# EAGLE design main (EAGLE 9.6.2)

## Sheet 1 of 4: Anschluesse
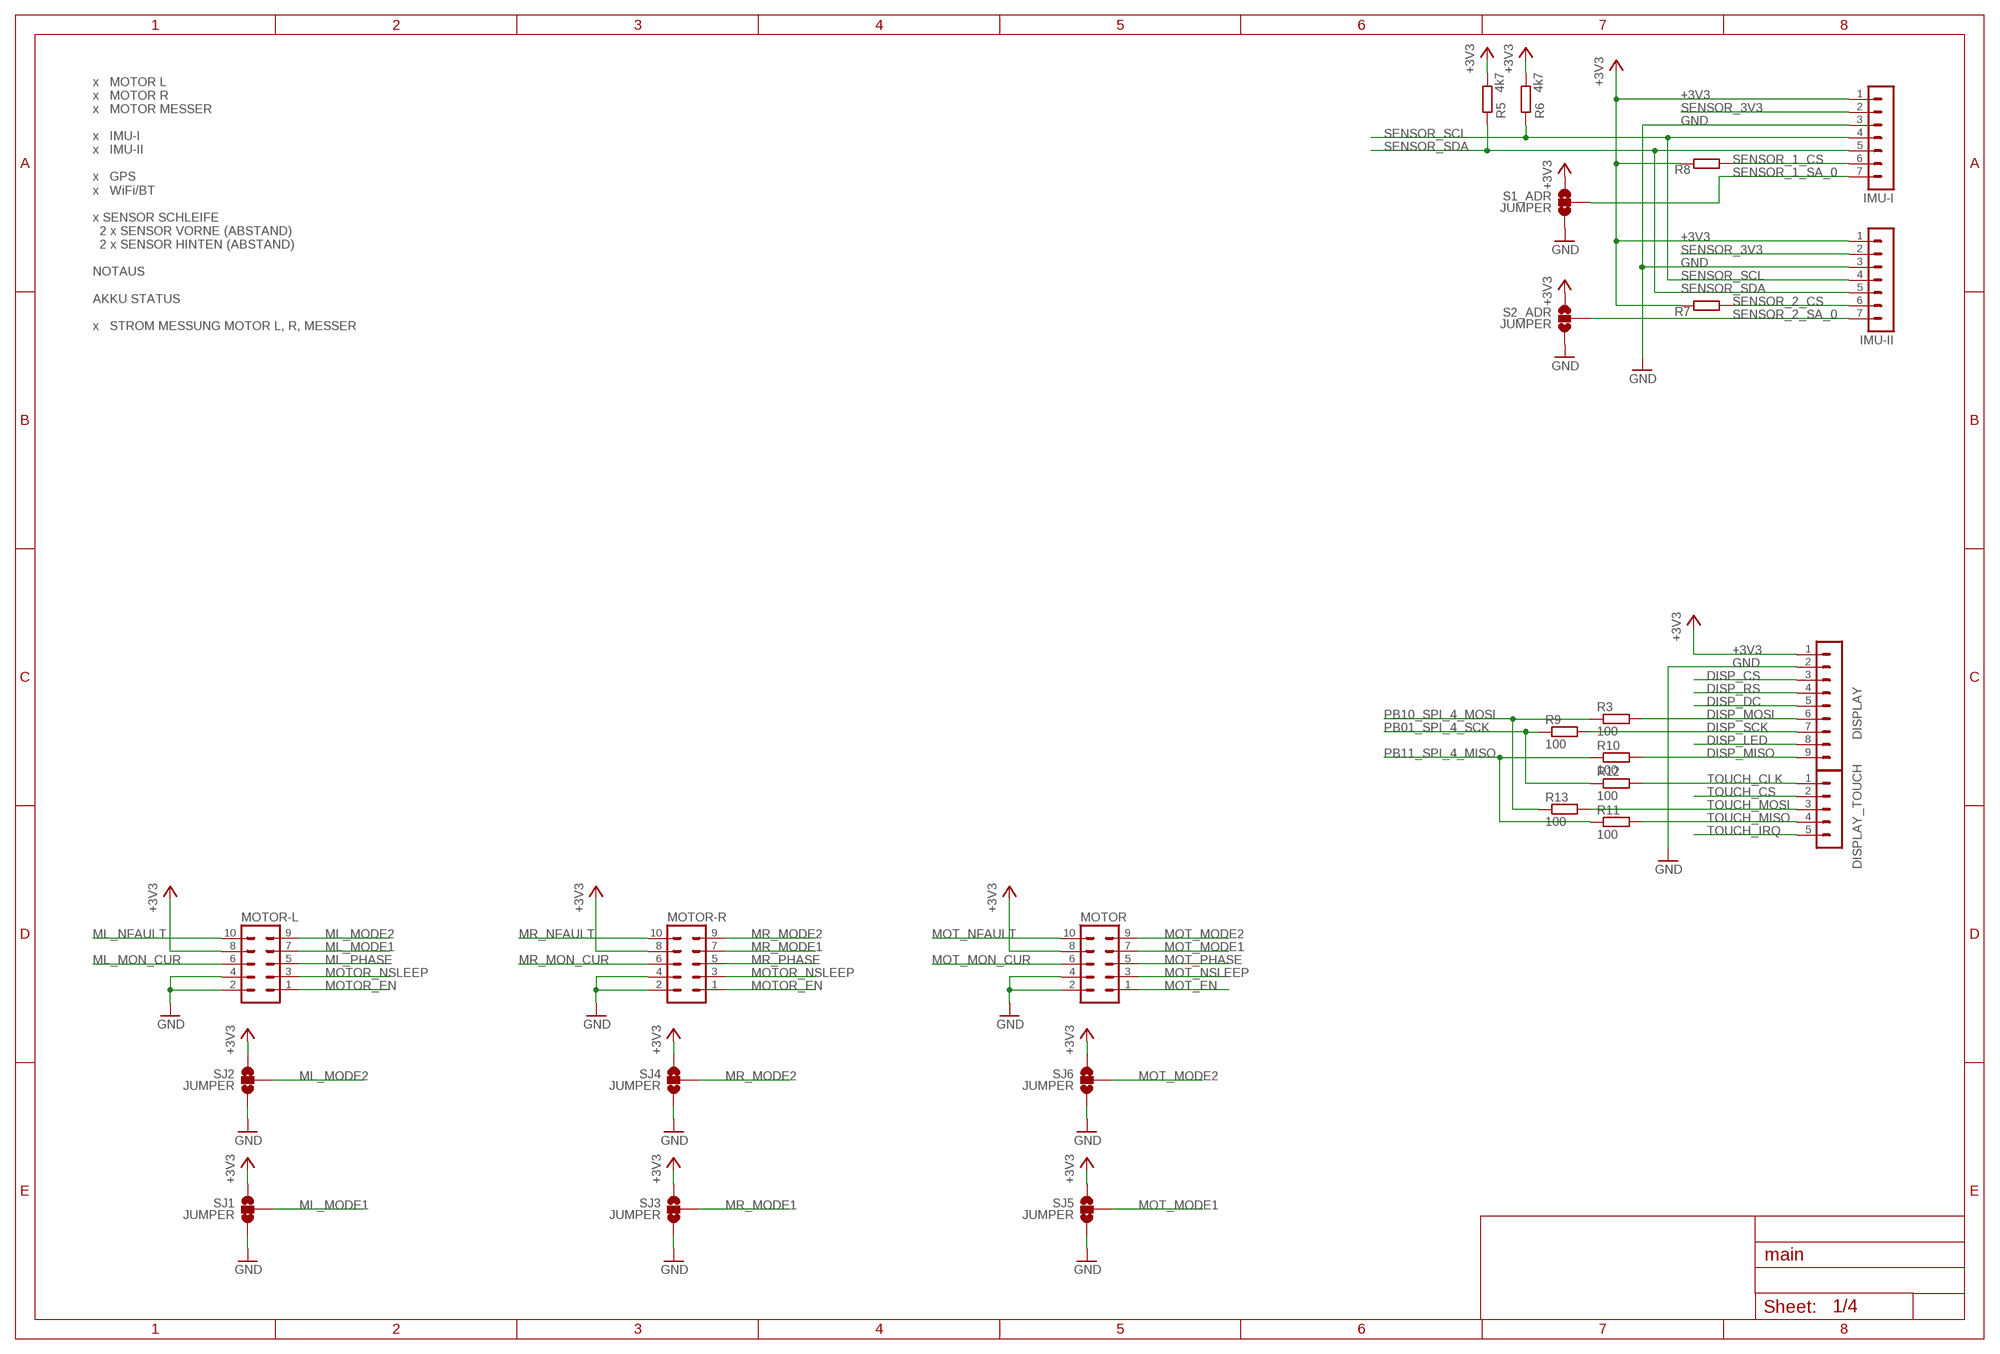
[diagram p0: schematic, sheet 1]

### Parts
DISPLAY  MA09-1  [MA09-1]
DISPLAY_TOUCH  MA05-1  [MA05-1]
IMU-I  MA07-1  [MA07-1]
IMU-II  MA07-1  [MA07-1]
MOTOR  ML10  [ML10]
MOTOR-L  ML10  [ML10]
MOTOR-R  ML10  [ML10]
R3  100  R-EU_R0603  [R0603]
R5  4k7  R-EU_R0603  [R0603]
R6  4k7  R-EU_R0603  [R0603]
R7  R-EU_R0603  [R0603]
R8  R-EU_R0603  [R0603]
R9  100  R-EU_R0603  [R0603]
R10  100  R-EU_R0603  [R0603]
R11  100  R-EU_R0603  [R0603]
R12  100  R-EU_R0603  [R0603]
R13  100  R-EU_R0603  [R0603]
S1_ADR  JUMPER  JUMPER-PAD-3-NOYES_SILK  [PAD-JUMPER-3-NO_YES_SILK]
S2_ADR  JUMPER  JUMPER-PAD-3-NOYES_SILK  [PAD-JUMPER-3-NO_YES_SILK]
SJ1  JUMPER  JUMPER-PAD-3-NOYES_SILK  [PAD-JUMPER-3-NO_YES_SILK]
SJ2  JUMPER  JUMPER-PAD-3-NOYES_SILK  [PAD-JUMPER-3-NO_YES_SILK]
SJ3  JUMPER  JUMPER-PAD-3-NOYES_SILK  [PAD-JUMPER-3-NO_YES_SILK]
SJ4  JUMPER  JUMPER-PAD-3-NOYES_SILK  [PAD-JUMPER-3-NO_YES_SILK]
SJ5  JUMPER  JUMPER-PAD-3-NOYES_SILK  [PAD-JUMPER-3-NO_YES_SILK]
SJ6  JUMPER  JUMPER-PAD-3-NOYES_SILK  [PAD-JUMPER-3-NO_YES_SILK]

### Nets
+3V3: DISPLAY.1 IMU-I.1 IMU-II.1 MOTOR-L.8 MOTOR-R.8 MOTOR.8 R5.2 R6.2 R7.2 R8.2 S1_ADR.1 S2_ADR.1 SJ1.1 SJ2.1 SJ3.1 SJ4.1 SJ5.1 SJ6.1 ; also sheet 2,3
DISP_CS: DISPLAY.3 ; also sheet 2
DISP_DC: DISPLAY.5 ; also sheet 2
DISP_LED: DISPLAY.8
DISP_MISO: DISPLAY.9 R10.2
DISP_MOSI: DISPLAY.6 R3.2
DISP_RS: DISPLAY.4 ; also sheet 2
DISP_SCK: DISPLAY.7 R9.2
GND: DISPLAY.2 IMU-I.3 IMU-II.3 MOTOR-L.2 MOTOR-L.4 MOTOR-R.2 MOTOR-R.4 MOTOR.2 MOTOR.4 S1_ADR.3 S2_ADR.3 SJ1.3 SJ2.3 SJ3.3 SJ4.3 SJ5.3 SJ6.3 ; also sheet 2,3,4
ML_MODE1: MOTOR-L.7 SJ1.2
ML_MODE2: MOTOR-L.9 SJ2.2
ML_MON_CUR: MOTOR-L.6 ; also sheet 2
ML_NFAULT: MOTOR-L.10 ; also sheet 2
ML_PHASE: MOTOR-L.5 ; also sheet 2
MOT_EN: MOTOR.1 ; also sheet 2
MOT_MODE1: MOTOR.7 SJ5.2
MOT_MODE2: MOTOR.9 SJ6.2
MOT_MON_CUR: MOTOR.6 ; also sheet 2
MOT_NFAULT: MOTOR.10 ; also sheet 2
MOT_NSLEEP: MOTOR.3 ; also sheet 2
MOT_PHASE: MOTOR.5 ; also sheet 2
MOTOR_EN: MOTOR-L.1 MOTOR-R.1 ; also sheet 2
MOTOR_NSLEEP: MOTOR-L.3 MOTOR-R.3 ; also sheet 2
MR_MODE1: MOTOR-R.7 SJ3.2
MR_MODE2: MOTOR-R.9 SJ4.2
MR_MON_CUR: MOTOR-R.6 ; also sheet 2
MR_NFAULT: MOTOR-R.10 ; also sheet 2
MR_PHASE: MOTOR-R.5 ; also sheet 2
PB01_SPI_4_SCK: R9.1 R12.1 ; also sheet 2
PB10_SPI_4_MOSI: R3.1 R13.1 ; also sheet 2
PB11_SPI_4_MISO: R10.1 R11.1 ; also sheet 2
SENSOR_1_CS: IMU-I.6 R8.1
SENSOR_1_SA_0: IMU-I.7 S1_ADR.2
SENSOR_2_CS: IMU-II.6 R7.1
SENSOR_2_SA_0: IMU-II.7 S2_ADR.2
SENSOR_3V3: IMU-I.2 IMU-II.2
SENSOR_SCL: IMU-I.4 IMU-II.4 R6.1 ; also sheet 2
SENSOR_SDA: IMU-I.5 IMU-II.5 R5.1 ; also sheet 2
TOUCH_CLK: DISPLAY_TOUCH.1 R12.2
TOUCH_CS: DISPLAY_TOUCH.2 ; also sheet 2
TOUCH_IRQ: DISPLAY_TOUCH.5 ; also sheet 2
TOUCH_MISO: DISPLAY_TOUCH.4 R11.2
TOUCH_MOSI: DISPLAY_TOUCH.3 R13.2

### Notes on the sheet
- x   MOTOR L
  x   MOTOR R
  x   MOTOR MESSER
  
  x   IMU-I
  x   IMU-II
  
  x   GPS
  x   WiFi/BT
  
  x SENSOR SCHLEIFE
    2 x SENSOR VORNE (ABSTAND)
    2 x SENSOR HINTEN (ABSTAND)
  
  NOTAUS
  
  AKKU STATUS
  
  x   STROM MESSUNG MOTOR L, R, MESSER

## Sheet 2 of 4: CPU
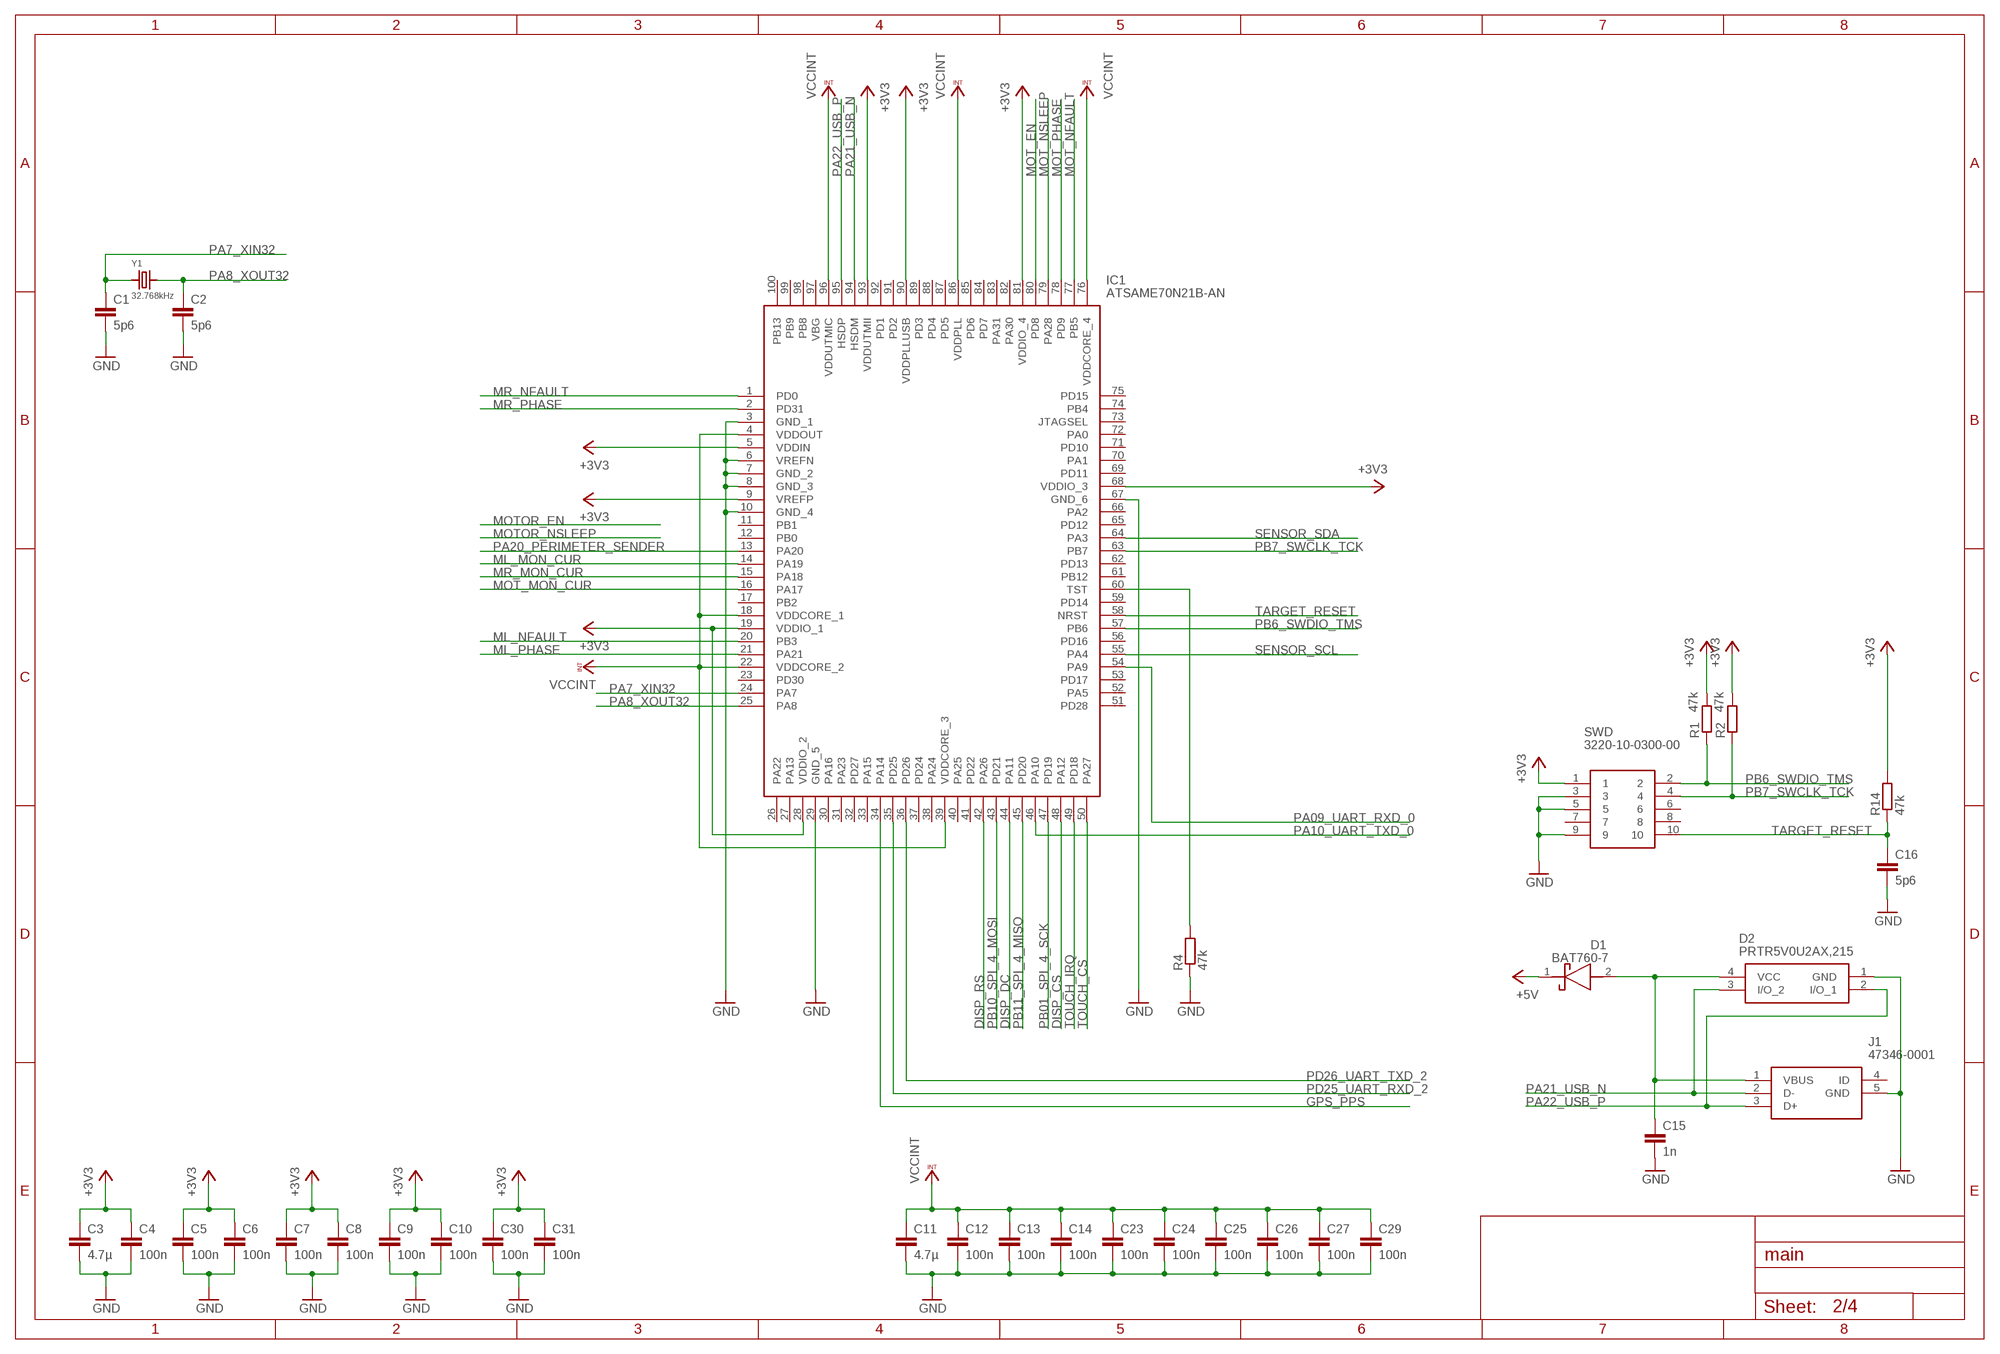
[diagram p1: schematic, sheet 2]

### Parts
C1  5p6  C-EUC0603  [C0603]
C2  5p6  C-EUC0603  [C0603]
C3  4.7µ  C-EUC0603  [C0603]
C4  100n  C-EUC0603  [C0603]
C5  100n  C-EUC0603  [C0603]
C6  100n  C-EUC0603  [C0603]
C7  100n  C-EUC0603  [C0603]
C8  100n  C-EUC0603  [C0603]
C9  100n  C-EUC0603  [C0603]
C10  100n  C-EUC0603  [C0603]
C11  4.7µ  C-EUC0603  [C0603]
C12  100n  C-EUC0603  [C0603]
C13  100n  C-EUC0603  [C0603]
C14  100n  C-EUC0603  [C0603]
C15  1n  C-EUC0603  [C0603]
C16  5p6  C-EUC0603  [C0603]
C23  100n  C-EUC0603  [C0603]
C24  100n  C-EUC0603  [C0603]
C25  100n  C-EUC0603  [C0603]
C26  100n  C-EUC0603  [C0603]
C27  100n  C-EUC0603  [C0603]
C29  100n  C-EUC0603  [C0603]
C30  100n  C-EUC0603  [C0603]
C31  100n  C-EUC0603  [C0603]
D1  BAT760-7  [SOD2513X120N]
D2  PRTR5V0U2AX,215  [PESD2ETHAXR]
IC1  ATSAME70N21B-AN  [QFP50P1600X1600X160-100N]
J1  47346-0001  [47346-0001]
R1  47k  R-EU_R0603  [R0603]
R2  47k  R-EU_R0603  [R0603]
R4  47k  R-EU_R0603  [R0603]
R14  47k  R-EU_R0603  [R0603]
SWD  3220-10-0300-00  [3220-10-0300-00]
Y1  32.768kHz  CRYSTALTHIN32K  [CRYSTAL_4.9X1.8]

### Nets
+3V3: C3.1 C4.1 C5.1 C6.1 C7.1 C8.1 C9.1 C10.1 C30.1 C31.1 IC1.5(VDDIN) IC1.9(VREFP) IC1.19(VDDIO_1) IC1.28(VDDIO_2) IC1.68(VDDIO_3) IC1.81(VDDIO_4) IC1.90(VDDPLLUSB) IC1.93(VDDUTMII) R1.2 R2.2 R14.2 SWD.1 ; also sheet 1,3
+5V: D1.1(K) ; also sheet 4
DISP_CS: IC1.48(PA12) ; also sheet 1
DISP_DC: IC1.44(PA11) ; also sheet 1
DISP_RS: IC1.42(PA26) ; also sheet 1
GND: C1.2 C2.2 C3.2 C4.2 C5.2 C6.2 C7.2 C8.2 C9.2 C10.2 C11.2 C12.2 C13.2 C14.2 C15.2 C16.2 C23.2 C24.2 C25.2 C26.2 C27.2 C29.2 C30.2 C31.2 D2.1(GND) IC1.3(GND_1) IC1.6(VREFN) IC1.7(GND_2) IC1.8(GND_3) IC1.10(GND_4) IC1.29(GND_5) IC1.67(GND_6) J1.5(GND) R4.1 SWD.3 SWD.5 SWD.9 ; also sheet 1,3,4
GPS_PPS: IC1.34(PA14) ; also sheet 3
ML_MON_CUR: IC1.14(PA19) ; also sheet 1
ML_NFAULT: IC1.20(PB3) ; also sheet 1
ML_PHASE: IC1.21(PA21) ; also sheet 1
MOT_EN: IC1.80(PD8) ; also sheet 1
MOT_MON_CUR: IC1.16(PA17) ; also sheet 1
MOT_NFAULT: IC1.77(PB5) ; also sheet 1
MOT_NSLEEP: IC1.79(PA28) ; also sheet 1
MOT_PHASE: IC1.78(PD9) ; also sheet 1
MR_MON_CUR: IC1.15(PA18) ; also sheet 1
MR_NFAULT: IC1.1(PD0) ; also sheet 1
MR_PHASE: IC1.2(PD31) ; also sheet 1
N$1: IC1.60(TST) R4.2
N$2: C15.1 D1.2(A) D2.4(VCC) J1.1(VBUS)
PA7_XIN32: C1.1 IC1.24(PA7) Y1.1
PA8_XOUT32: C2.1 IC1.25(PA8) Y1.2
PA09_UART_RXD_0: IC1.54(PA9) ; also sheet 3
PA10_UART_TXD_0: IC1.46(PA10) ; also sheet 3
PA20_PERIMETER_SENDER: IC1.13(PA20) ; also sheet 4
PA21_USB_N: D2.3(I/O_2) IC1.94(HSDM) J1.2(D-)
PA22_USB_P: D2.2(I/O_1) IC1.95(HSDP) J1.3(D+)
PB01_SPI_4_SCK: IC1.47(PD19) ; also sheet 1
PB6_SWDIO_TMS: IC1.57(PB6) R1.1 SWD.2
PB7_SWCLK_TCK: IC1.63(PB7) R2.1 SWD.4
PB10_SPI_4_MOSI: IC1.43(PD21) ; also sheet 1
PB11_SPI_4_MISO: IC1.45(PD20) ; also sheet 1
PD25_UART_RXD_2: IC1.35(PD25) ; also sheet 3
PD26_UART_TXD_2: IC1.36(PD26) ; also sheet 3
SENSOR_SCL: IC1.55(PA4) ; also sheet 1
SENSOR_SDA: IC1.64(PA3) ; also sheet 1
TARGET_RESET: C16.1 IC1.58(NRST) R14.1 SWD.10
TOUCH_CS: IC1.50(PA27) ; also sheet 1
TOUCH_IRQ: IC1.49(PD18) ; also sheet 1
VCCINT: C11.1 C12.1 C13.1 C14.1 C23.1 C24.1 C25.1 C26.1 C27.1 C29.1 IC1.4(VDDOUT) IC1.18(VDDCORE_1) IC1.22(VDDCORE_2) IC1.39(VDDCORE_3) IC1.76(VDDCORE_4) IC1.86(VDDPLL) IC1.96(VDDUTMIC)
Unconnected: IC1.11(PB1) IC1.12(PB0) IC1.17(PB2) IC1.23(PD30) IC1.26(PA22) IC1.27(PA13) IC1.30(PA16) IC1.31(PA23) IC1.32(PD27) IC1.33(PA15) IC1.37(PD24) IC1.38(PA24) IC1.40(PA25) IC1.41(PD22) IC1.51(PD28) IC1.52(PA5) IC1.53(PD17) IC1.56(PD16) IC1.59(PD14) IC1.61(PB12) IC1.62(PD13) IC1.65(PD12) IC1.66(PA2) IC1.69(PD11) IC1.70(PA1) IC1.71(PD10) IC1.72(PA0) IC1.73(JTAGSEL) IC1.74(PB4) IC1.75(PD15) IC1.82(PA30) IC1.83(PA31) IC1.84(PD7) IC1.85(PD6) IC1.87(PD5) IC1.88(PD4) IC1.89(PD3) IC1.91(PD2) IC1.92(PD1) IC1.97(VBG) IC1.98(PB8) IC1.99(PB9) IC1.100(PB13) J1.4(ID) SWD.6 SWD.7 SWD.8

## Sheet 3 of 4: GPS WLAN BT
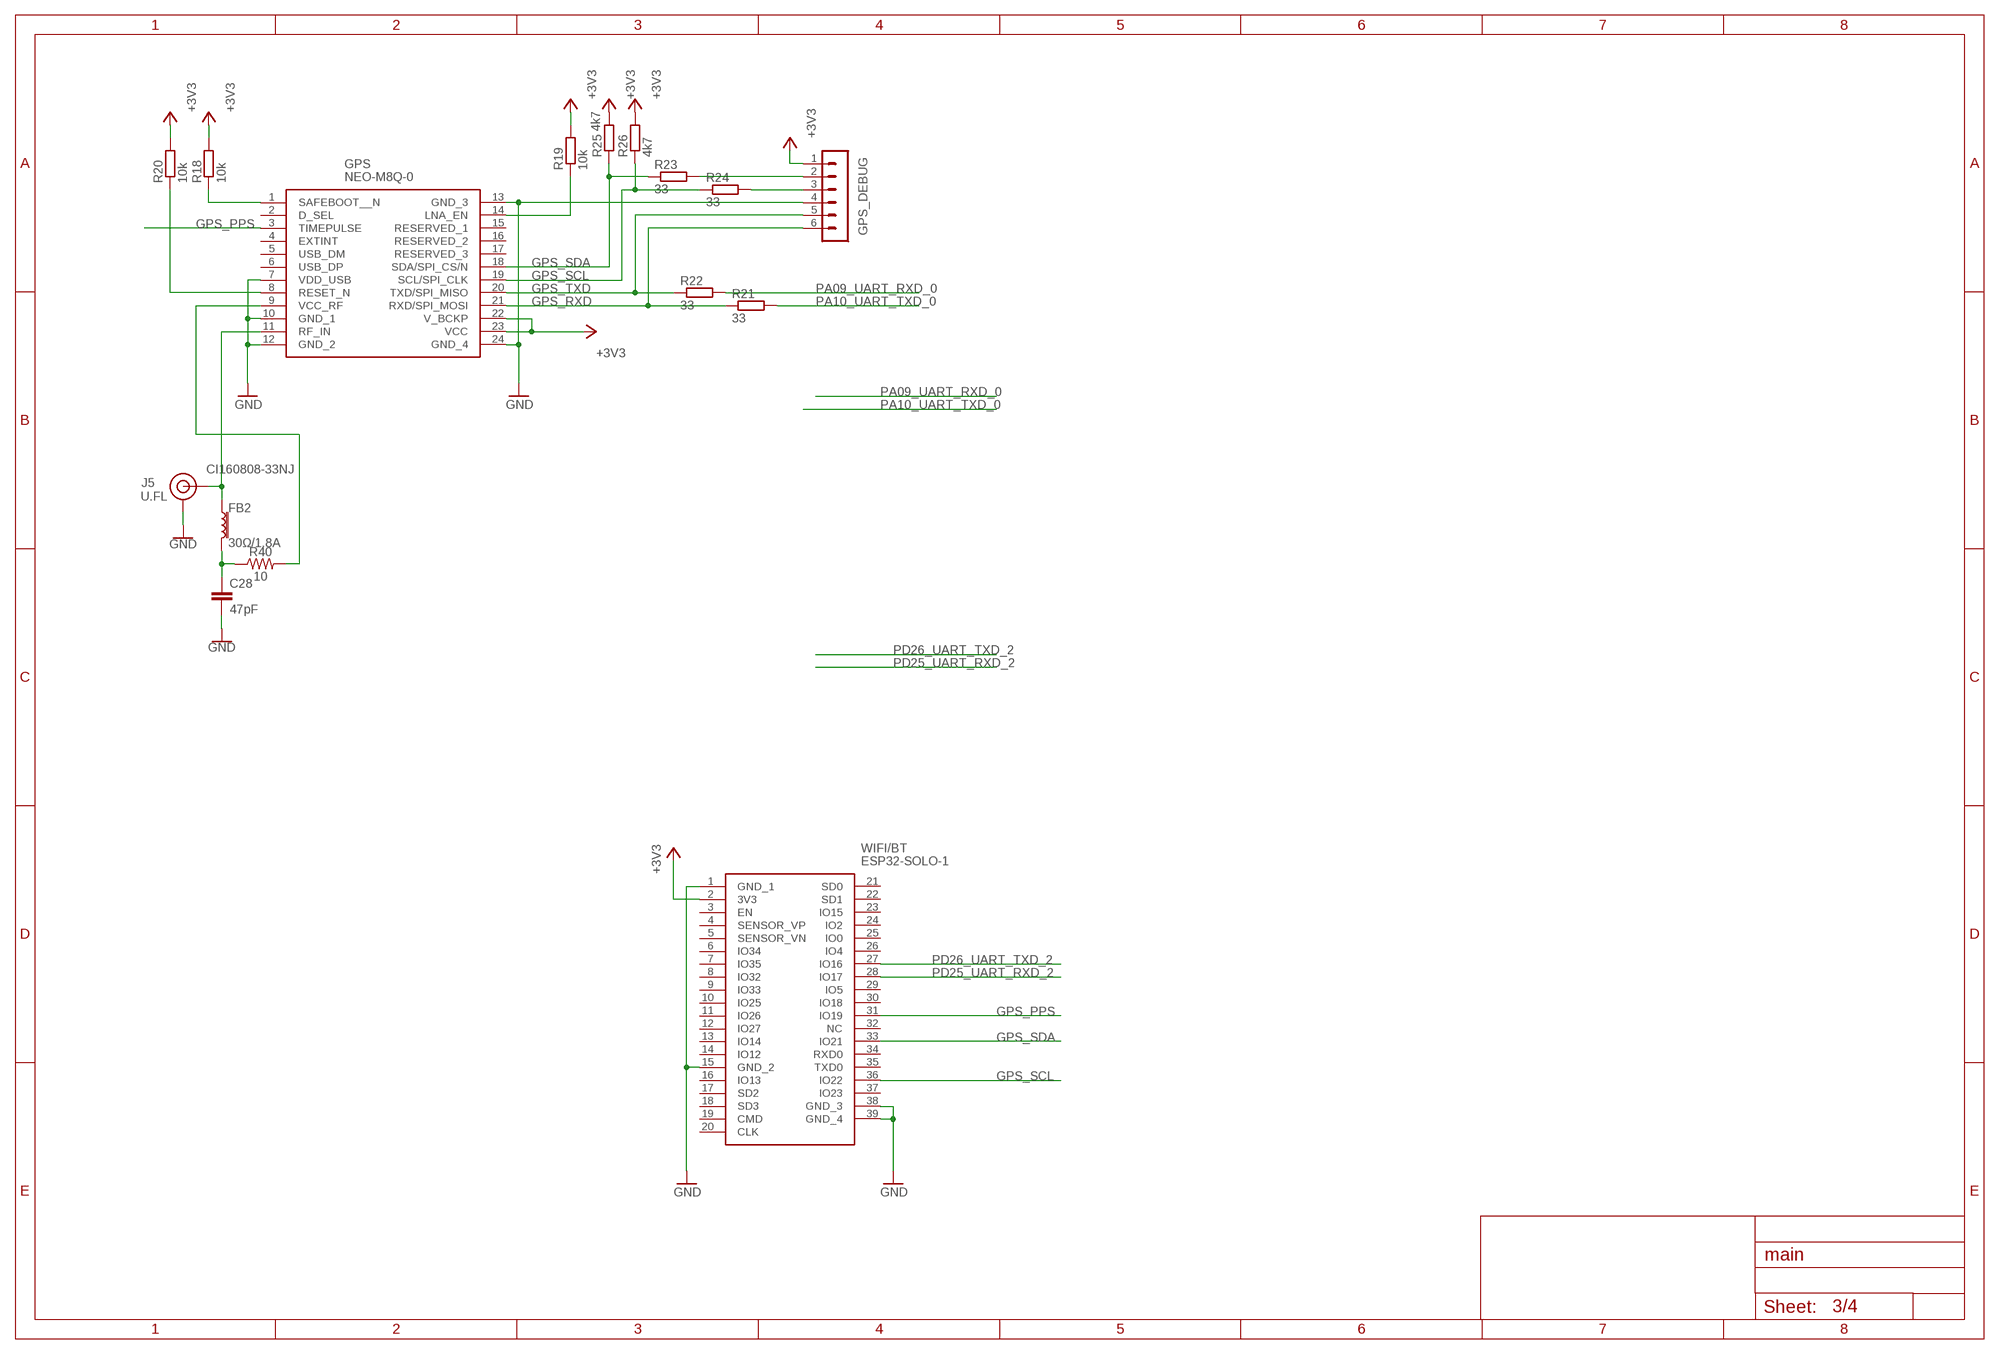
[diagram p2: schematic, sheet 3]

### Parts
C28  47pF  47PF-0603-50V-5%  [0603]
FB2  30Ω/1.8A  FERRITE_BEAD-0603  [0603]
GPS  NEO-M8Q-0  [NEO-M8U]
GPS_DEBUG  MA06-1  [MA06-1]
J5  U.FL  U.FL2PIN  [U.FL]
R18  10k  R-EU_R0603  [R0603]
R19  10k  R-EU_R0603  [R0603]
R20  10k  R-EU_R0603  [R0603]
R21  33  R-EU_R0603  [R0603]
R22  33  R-EU_R0603  [R0603]
R23  33  R-EU_R0603  [R0603]
R24  33  R-EU_R0603  [R0603]
R25  4k7  R-EU_R0603  [R0603]
R26  4k7  R-EU_R0603  [R0603]
R40  10  10OHM-0603-1/10W-1%  [0603]
WIFI/BT  ESP32-SOLO-1  [ESP32SOLO1]

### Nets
+3V3: GPS.22(V_BCKP) GPS.23(VCC) GPS_DEBUG.1 R18.2 R19.2 R20.2 R25.2 R26.2 WIFI/BT.2(3V3) ; also sheet 1,2
ANT_VCC1: C28.1 FB2.2 R40.1
GND: C28.2 GPS.7(VDD_USB) GPS.10(GND_1) GPS.12(GND_2) GPS.13(GND_3) GPS.24(GND_4) GPS_DEBUG.4 J5.1(GND) J5.2(GND) WIFI/BT.1(GND_1) WIFI/BT.15(GND_2) WIFI/BT.38(GND_3) WIFI/BT.39(GND_4) ; also sheet 1,2,4
GPS_ANT2: FB2.1 GPS.11(RF_IN) J5.FEED(SIGNAL)
GPS_PPS: GPS.3(TIMEPULSE) WIFI/BT.31(IO19) ; also sheet 2
GPS_RXD: GPS.21(RXD/SPI_MOSI) GPS_DEBUG.6 R21.1
GPS_SCL: GPS.19(SCL/SPI_CLK) R24.1 R26.1 WIFI/BT.36(IO22)
GPS_SDA: GPS.18(SDA/SPI_CS/N) R23.1 R25.1 WIFI/BT.33(IO21)
GPS_TXD: GPS.20(TXD/SPI_MISO) GPS_DEBUG.5 R22.1
N$5: GPS_DEBUG.2 R23.2
N$12: GPS_DEBUG.3 R24.2
N$13: GPS.1(SAFEBOOT__N) R18.1
N$14: GPS.8(RESET_N) R20.1
N$15: GPS.14(LNA_EN) R19.1
N$29: GPS.9(VCC_RF) R40.2
PA09_UART_RXD_0: R22.2 ; also sheet 2
PA10_UART_TXD_0: R21.2 ; also sheet 2
PD25_UART_RXD_2: WIFI/BT.28(IO17) ; also sheet 2
PD26_UART_TXD_2: WIFI/BT.27(IO16) ; also sheet 2
Unconnected: GPS.2(D_SEL) GPS.4(EXTINT) GPS.5(USB_DM) GPS.6(USB_DP) GPS.15(RESERVED_1) GPS.16(RESERVED_2) GPS.17(RESERVED_3) WIFI/BT.3(EN) WIFI/BT.4(SENSOR_VP) WIFI/BT.5(SENSOR_VN) WIFI/BT.6(IO34) WIFI/BT.7(IO35) WIFI/BT.8(IO32) WIFI/BT.9(IO33) WIFI/BT.10(IO25) WIFI/BT.11(IO26) WIFI/BT.12(IO27) WIFI/BT.13(IO14) WIFI/BT.14(IO12) WIFI/BT.16(IO13) WIFI/BT.17(SD2) WIFI/BT.18(SD3) WIFI/BT.19(CMD) WIFI/BT.20(CLK) WIFI/BT.21(SD0) WIFI/BT.22(SD1) WIFI/BT.23(IO15) WIFI/BT.24(IO2) WIFI/BT.25(IO0) WIFI/BT.26(IO4) WIFI/BT.29(IO5) WIFI/BT.30(IO18) WIFI/BT.32(NC) WIFI/BT.34(RXD0) WIFI/BT.35(TXD0) WIFI/BT.37(IO23)

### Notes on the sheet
- CI160808-33NJ

## Sheet 4 of 4: POWER
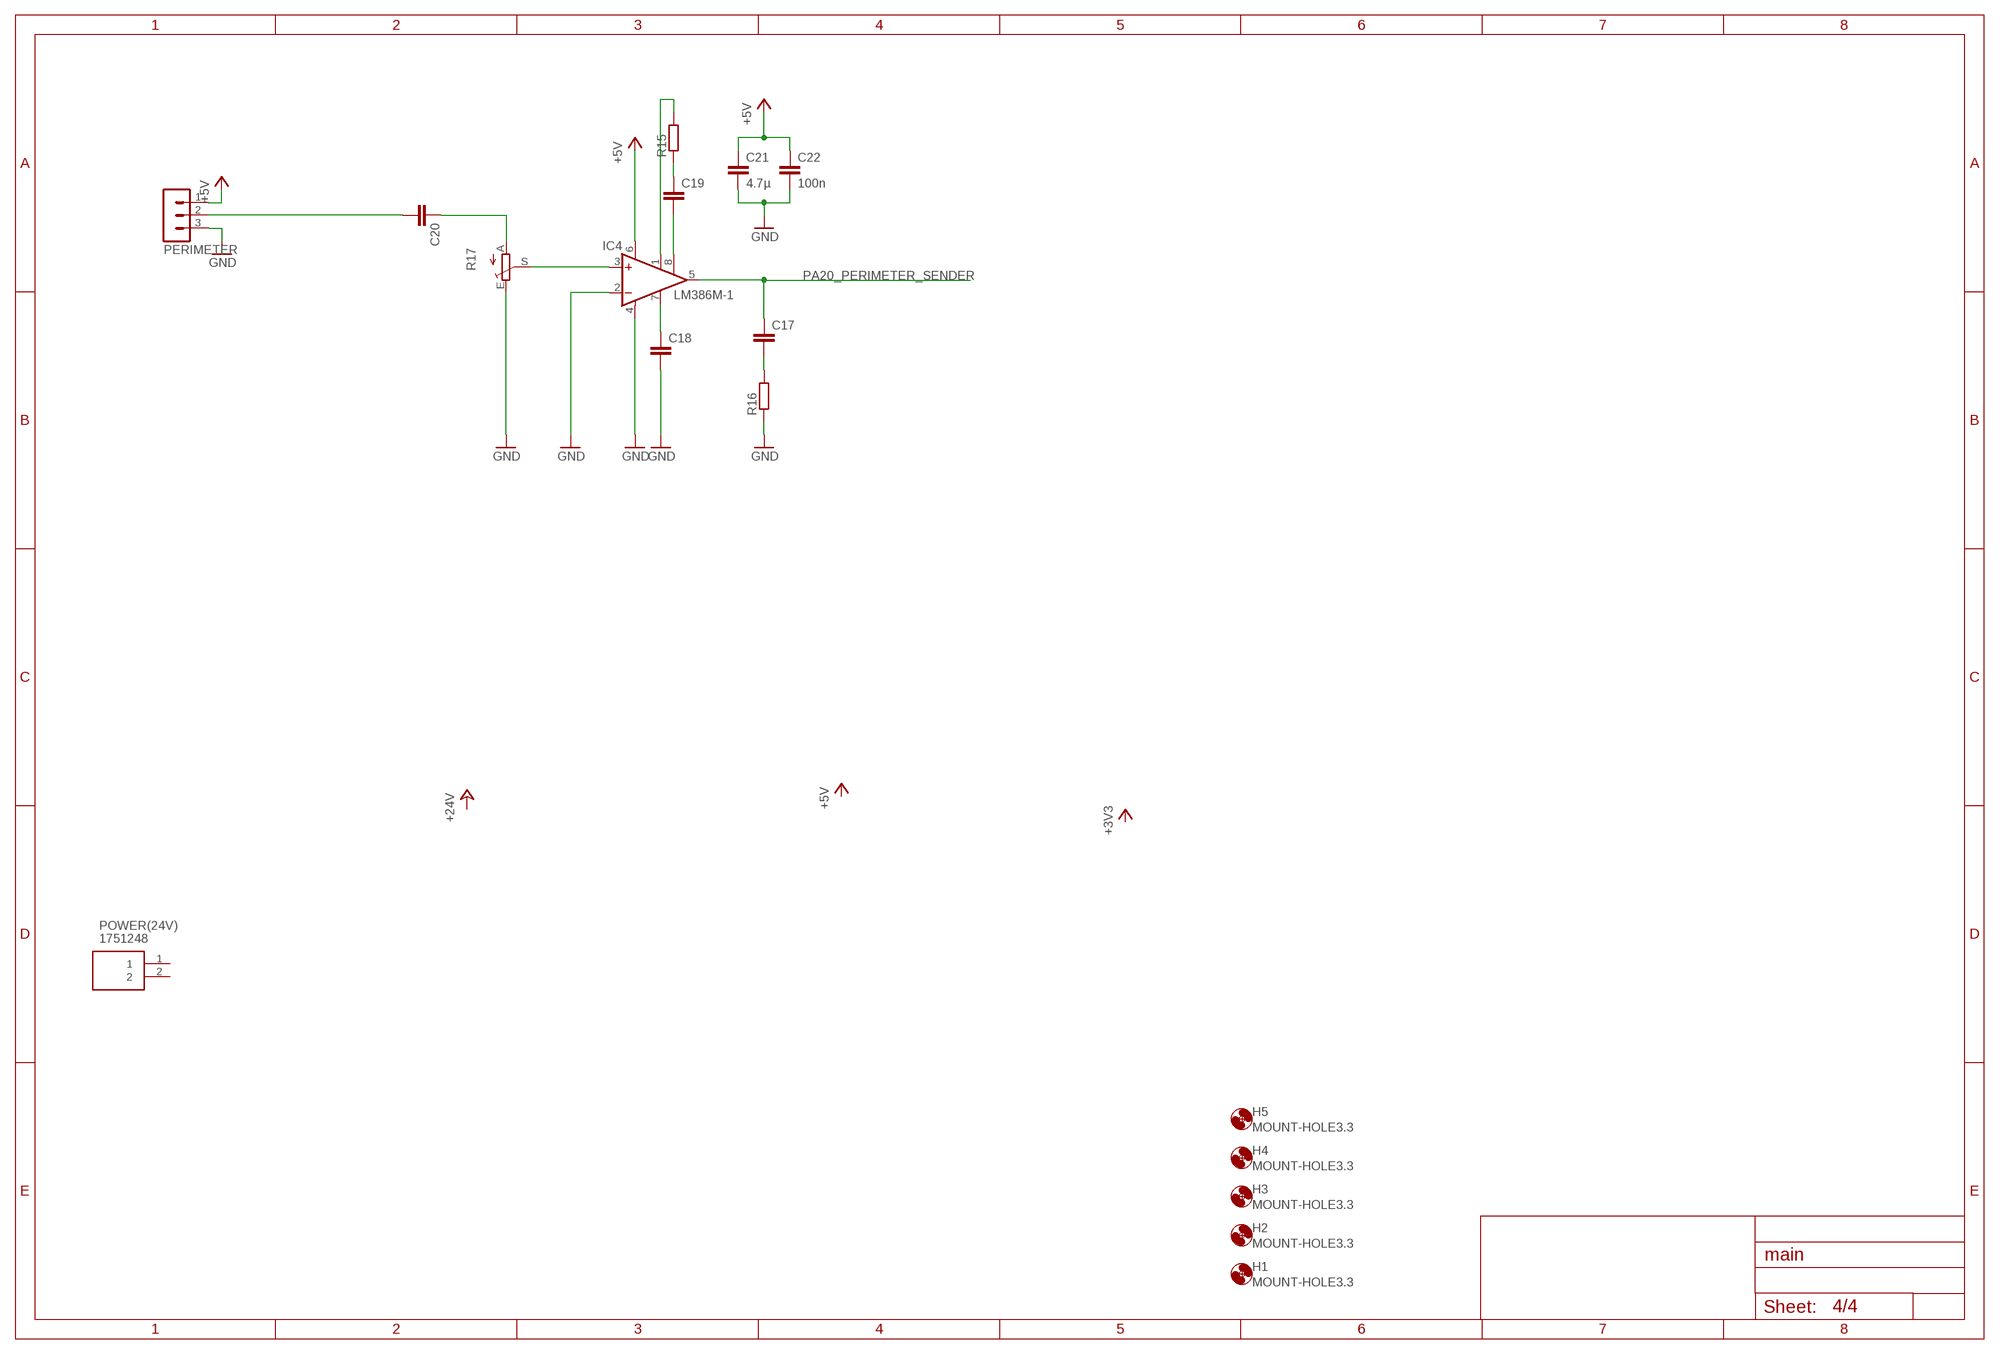
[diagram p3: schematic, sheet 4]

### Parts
C17  C-EUC0603  [C0603]
C18  C-EUC0603  [C0603]
C19  C-EUC0603  [C0603]
C20  C-EUC0603  [C0603]
C21  4.7µ  C-EUC0603  [C0603]
C22  100n  C-EUC0603  [C0603]
H1  MOUNT-HOLE3.3  [3,3]
H2  MOUNT-HOLE3.3  [3,3]
H3  MOUNT-HOLE3.3  [3,3]
H4  MOUNT-HOLE3.3  [3,3]
H5  MOUNT-HOLE3.3  [3,3]
IC4  LM386M-1  [SO08]
PERIMETER  MA03-1  [MA03-1]
POWER(24V)  1751248  [SHDR2W90P0X350_1X2_750X730X850]
R15  R-EU_R0603  [R0603]
R16  R-EU_R0603  [R0603]
R17  TRIM_1234-S64YW  [S64YW]

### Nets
+5V: C21.1 C22.1 IC4.6(VS) PERIMETER.1 ; also sheet 2
GND: C18.2 C21.2 C22.2 IC4.2(-IN) IC4.4(GND) PERIMETER.3 R16.1 R17.E ; also sheet 1,2,3
N$3: C18.1 IC4.7(BYPASS)
N$4: C17.2 R16.2
N$6: C19.2 IC4.8(GAIN)
N$7: IC4.1(GAIN) R15.2
N$8: C19.1 R15.1
N$9: C20.1 R17.A
N$10: IC4.3(+IN) R17.S
N$11: C20.2 PERIMETER.2
PA20_PERIMETER_SENDER: C17.1 IC4.5(OUT) ; also sheet 2
Unconnected: POWER(24V).1 POWER(24V).2 R17.S@1(S)

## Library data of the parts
C1-C27 C29-C31 = rcl:C-EU: CAPACITOR, European symbol; SPICEPREFIX: C
C28 = SparkFun-Capacitors:47PF: 47pF ceramic capacitors; PROD_ID: CAP-08913
D1 = SamacSys_Parts:BAT760-7: Diode Schottky 30V 1A 2Pin SOD323 Diodes Inc BAT760-7, SMT Schottky Diode, 30V 1A, 2-Pin SOD-323; ARROW_PART_NUMBER: BAT760-7; ARROW_PRICE-STOCK: https://www.arrow.com/en/products/bat760-7/diodes-incorporated; DESCRIPTION: Diode Schottky 30V 1A 2Pin SOD323 Diodes Inc BAT760-7, SMT Schottky Diode, 30V 1A, 2-Pin SOD-323; HEIGHT: 1.2mm; MANUFACTURER_NAME: Diodes Inc.; MANUFACTURER_PART_NUMBER: BAT760-7; MOUSER_PART_NUMBER: 621-BAT760-7; MOUSER_PRICE-STOCK: https://www.mouser.co.uk/ProductDetail/Diodes-Incorporated/BAT760-7?qs=JV7lzlMm3yKDDyO09xoRbQ%3D%3D
D2 = SamacSys_Parts:PRTR5V0U2AX,215: Nexperia PRTR5V0U2AX,215, Dual Uni-Directional TVS Diode, 4-Pin SOT-143B Source: Datasheet; ARROW_PART_NUMBER: PRTR5V0U2AX,215; ARROW_PRICE-STOCK: https://www.arrow.com/en/products/prtr5v0u2ax215/nexperia; DESCRIPTION: Nexperia PRTR5V0U2AX,215, Dual Uni-Directional TVS Diode, 4-Pin SOT-143B; HEIGHT: 1mm; MANUFACTURER_NAME: Nexperia; MANUFACTURER_PART_NUMBER: PRTR5V0U2AX,215; MOUSER_PART_NUMBER: 771-PRTR5V0U2AX-T/R; MOUSER_PRICE-STOCK: https://www.mouser.co.uk/ProductDetail/Nexperia/PRTR5V0U2AX215?qs=LOCUfHb8d9sgAt584ov2VQ%3D%3D
DISPLAY = con-lstb:MA09-1: PIN HEADER; OC_FARNELL: unknown; OC_NEWARK: unknown
DISPLAY_TOUCH = con-lstb:MA05-1: PIN HEADER; OC_FARNELL: unknown; OC_NEWARK: unknown
FB2 = SparkFun-Coils:FERRITE_BEAD: Ferrite Bead (blocks, cores, rings, chokes, etc.); PROD_ID: NDUC-13805
GPS = SamacSys_Parts:NEO-M8Q-0: NEO-M8 RF Receiver BeiDou, Galileo, GLONASS, GNSS, GPS 1.575GHz -167dBm Source: Datasheet; DESCRIPTION: NEO-M8 RF Receiver BeiDou, Galileo, GLONASS, GNSS, GPS 1.575GHz -167dBm; HEIGHT: mm; MANUFACTURER_NAME: U-Blox; MANUFACTURER_PART_NUMBER: NEO-M8Q-0
GPS_DEBUG = con-lstb:MA06-1: PIN HEADER; OC_FARNELL: unknown; OC_NEWARK: unknown
H1-H5 = holes:MOUNT-HOLE: MOUNTING HOLE with drill center marker
IC1 = SamacSys_Parts:ATSAME70N21B-AN: Microchip ATSAME70N21B-AN, 32bit ARM Cortex M7 Microcontroller, 300MHz, 2 MB Flash, 100-Pin LQFP Source: Datasheet; ARROW_PART_NUMBER: ATSAME70N21B-AN; ARROW_PRICE-STOCK: https://www.arrow.com/en/products/atsame70n21b-an/microchip-technology; DESCRIPTION: Microchip ATSAME70N21B-AN, 32bit ARM Cortex M7 Microcontroller, 300MHz, 2 MB Flash, 100-Pin LQFP; HEIGHT: 1.6mm; MANUFACTURER_NAME: Microchip; MANUFACTURER_PART_NUMBER: ATSAME70N21B-AN; MOUSER_PART_NUMBER: 556-ATSAME70N21B-AN; MOUSER_PRICE-STOCK: https://www.mouser.co.uk/ProductDetail/Microchip-Technology/ATSAME70N21B-AN?qs=chTDxNqvsymrWo89LU8OYw%3D%3D
IC4 = linear:LM386?-*: Low Voltage Audio Power Amplifier Source: http://cache.national.com/ds/LM/LM386.pdf
IMU-I IMU-II = con-lstb:MA07-1: PIN HEADER; OC_FARNELL: unknown; OC_NEWARK: unknown
J1 = SamacSys_Parts:47346-0001: Micro USB B Receptacle Bottom Mount Assy Molex Right Angle SMT Type B Version 2.0 Micro USB Connector Socket, 30 V ac, 1A 47352 MICRO-USB Source: Datasheet; ARROW_PART_NUMBER: 47346-0001; DESCRIPTION: Micro USB B Receptacle Bottom Mount Assy Molex Right Angle SMT Type B Version 2.0 Micro USB Connector Socket, 30 V ac, 1A 47352 MICRO-USB; HEIGHT: mm; MANUFACTURER_NAME: Molex; MANUFACTURER_PART_NUMBER: 47346-0001; MOUSER_PART_NUMBER: 538-47346-0001; MOUSER_PRICE-STOCK: https://www.mouser.co.uk/ProductDetail/Molex/47346-0001?qs=c2CV6XM0DweJBWaSeyWeCw%3D%3D
J5 = SparkFun-Connectors:U.FL2PIN: SMD Antenna Connector - U.FL; PROD_ID: CONN-09193; SF_ID: WRL-09144
MOTOR MOTOR-L MOTOR-R = con-ml:ML10: HARTING; OC_FARNELL: unknown; OC_NEWARK: unknown
PERIMETER = con-lstb:MA03-1: PIN HEADER; OC_FARNELL: unknown; OC_NEWARK: unknown
POWER(24V) = SamacSys_Parts:1751248: PCB terminal block, 3.5mm pitch, 2 way Phoenix Contact COMBICON MKDS Series 3.5mm Pitch Straight PCB Terminal Block with Screw Termination, Through Hole; ALLIED_NUMBER: 70054346; ALLIED_PRICE-STOCK: https://www.alliedelec.com/phoenix-contact-1751248/70054346/; DESCRIPTION: PCB terminal block, 3.5mm pitch, 2 way Phoenix Contact COMBICON MKDS Series 3.5mm Pitch Straight PCB Terminal Block with Screw Termination, Through Hole; HEIGHT: 8.5mm; MANUFACTURER_NAME: Phoenix Contact; MANUFACTURER_PART_NUMBER: 1751248; MOUSER_PART_NUMBER: 651-1751248; MOUSER_PRICE-STOCK: https://www.mouser.com/Search/Refine.aspx?Keyword=651-1751248; RS_PART_NUMBER: 8024849; RS_PRICE-STOCK: http://uk.rs-online.com/web/p/products/8024849
R1-R16 R18-R26 = rcl:R-EU_: RESISTOR, European symbol; SPICEPREFIX: R
R17 = pot:TRIM_1234-: POTENTIOMETER
R40 = SparkFun-Resistors:10OHM: 10Ω resistor; PROD_ID: RES-12581
S1_ADR S2_ADR SJ1-SJ6 = SparkFun-Connectors:JUMPER-PAD-3-NO
SWD = SamacSys_Parts:3220-10-0300-00: IDC BOX HEADER 0.050 10 POS Source: Datasheet; DESCRIPTION: IDC BOX HEADER 0.050 10 POS; HEIGHT: mm; MANUFACTURER_NAME: CNC Tech; MANUFACTURER_PART_NUMBER: 3220-10-0300-00
WIFI/BT = SamacSys_Parts:ESP32-SOLO-1: WiFi Modules (802.11) SMD Module, ESP32-S0WD, 32Mbits SPI flash, UART mode, PCB antenna Source: Datasheet; DESCRIPTION: WiFi Modules (802.11) SMD Module, ESP32-S0WD, 32Mbits SPI flash, UART mode, PCB antenna; HEIGHT: 3.1mm; MANUFACTURER_NAME: Espressif; MANUFACTURER_PART_NUMBER: ESP32-SOLO-1; MOUSER_PART_NUMBER: 356-ESP32-SOLO-1
Y1 = microbuilder:CRYSTAL: Crystals

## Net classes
2 3.3V: width 0.508 mm

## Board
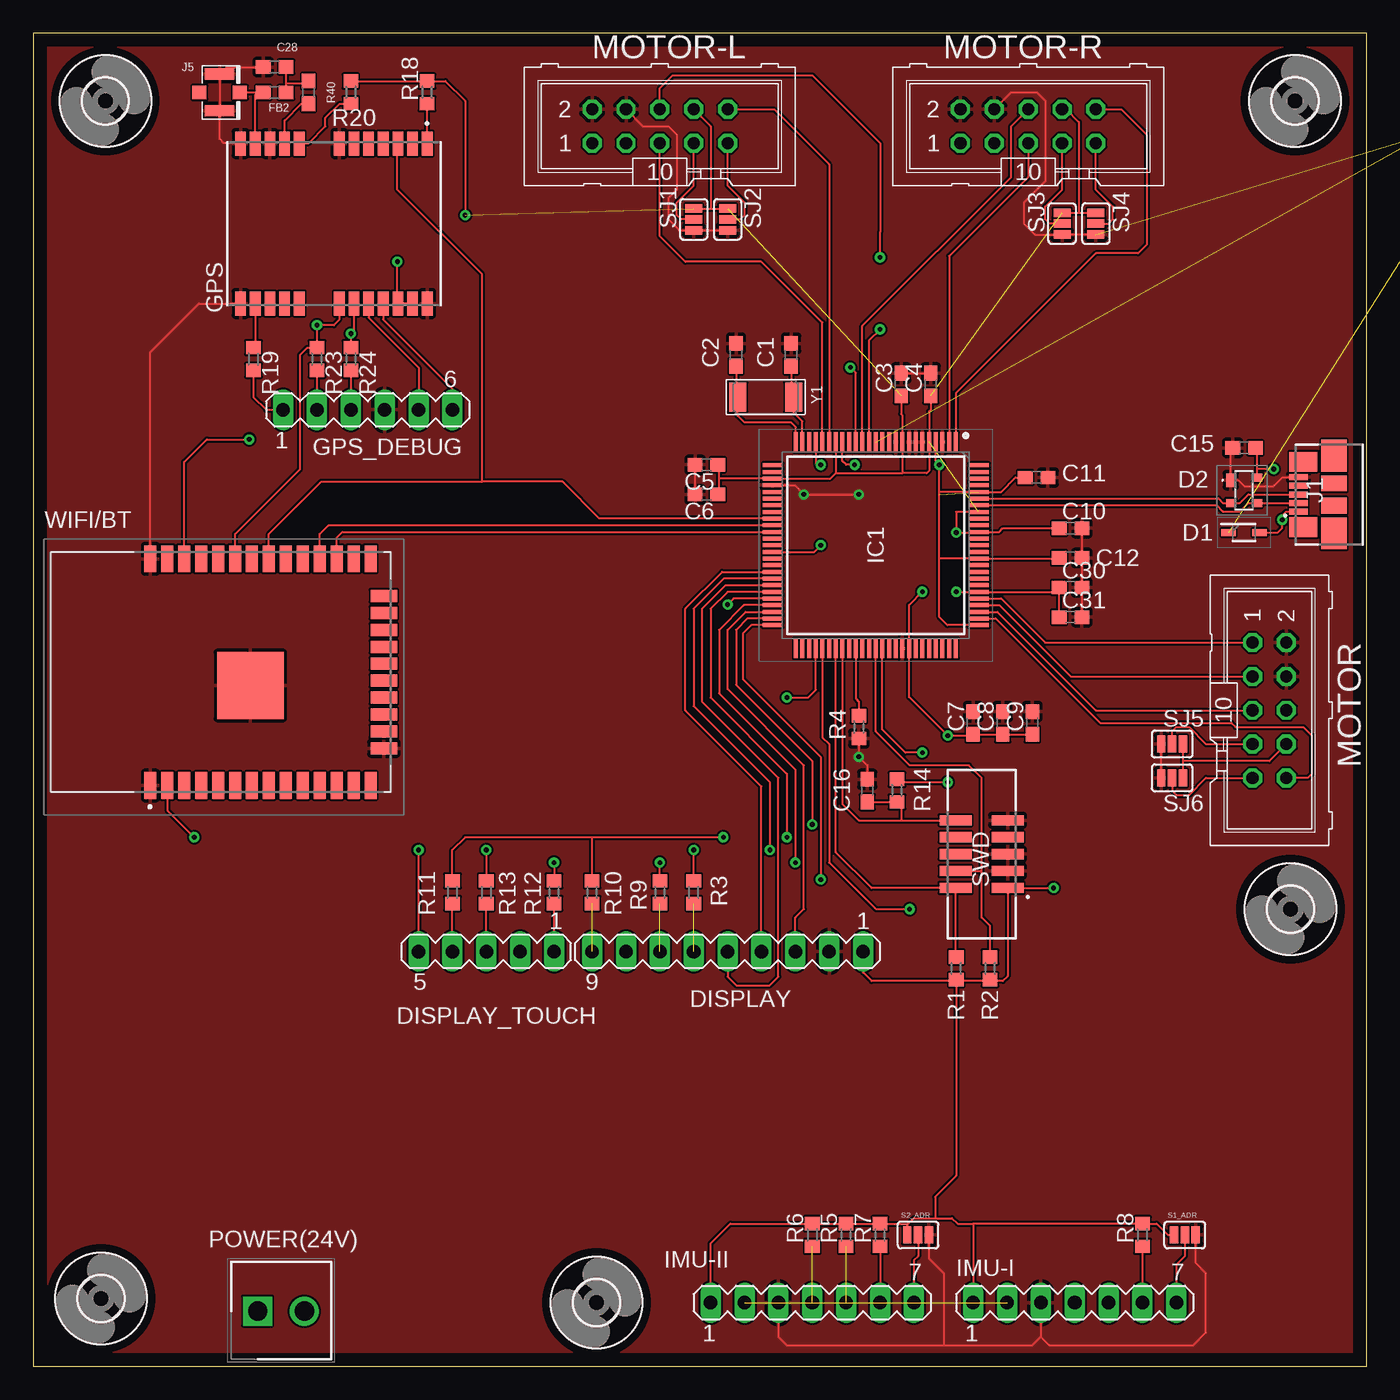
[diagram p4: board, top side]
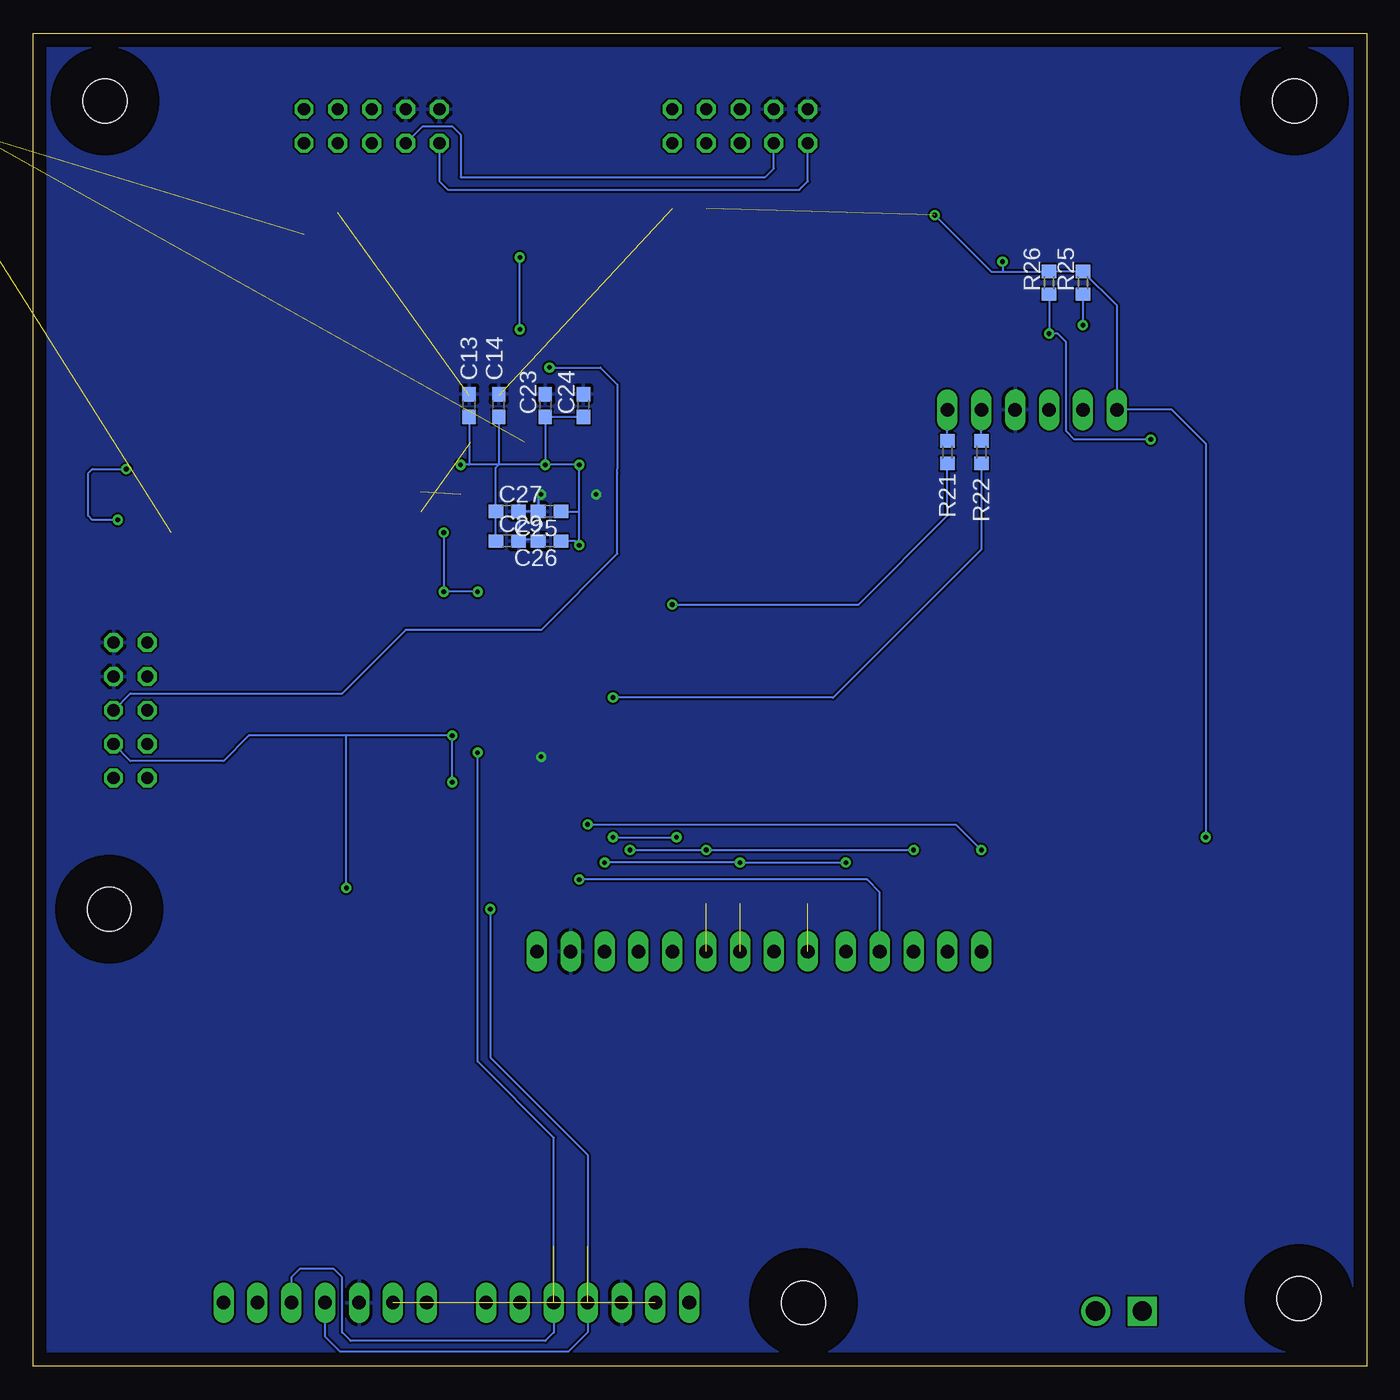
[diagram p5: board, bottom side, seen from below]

Size 99.99 x 100 mm. Coordinates in mm from the lower left corner, seen from the top.
Outline: 0,0 99.99,0 99.99,100 0,100 0,0
Copper layers (1*16): Top 0.035mm / dielectric 1.5mm / Bottom 0.035mm
Design rules "default": minimum track width 6mil, minimum drill 0.35mm, track to track 6mil, track to pad 6mil, pad to pad 6mil, via to via 6mil, smd to smd 6mil, copper to edge 40mil, drill to drill 6mil, minimum pad ring 10mil, minimum via ring 8mil, stop-mask expansion 4mil, vias tented up to drill 0mil, thermal gap 10mil

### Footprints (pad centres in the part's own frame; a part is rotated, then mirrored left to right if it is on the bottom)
C0603 = smd 1.1 x 1: 1 -0.85,0; 2 0.85,0
0603 = smd 1.1 x 1: 1 -0.85,0; 2 0.85,0
SOD2513X120N = smd 1.075 x 0.5: 1 -1.162,0; 2 1.162,0
PESD2ETHAXR = smd 1 x 0.7: 1 -0.75,-1 | smd 0.6 x 0.7: 2 0.95,-1; 3 0.95,1; 4 -0.95,1
MA09-1 = drill 1.016 long: 1 -10.16,0; 2 -7.62,0; 3 -5.08,0; 4 -2.54,0; 5 0,0; 6 2.54,0; 7 5.08,0; 8 7.62,0; 9 10.16,0
MA05-1 = drill 1.016 long: 1 -5.08,0; 2 -2.54,0; 3 0,0; 4 2.54,0; 5 5.08,0
NEO-M8U = smd 1.8 x 0.8: 1 6,-7; 2 6,-5.9; 3 6,-4.8; 4 6,-3.7; 5 6,-2.6; 6 6,-1.5; 7 6,-0.4; 8 6,2.6; 9 6,3.7; 10 6,4.8; 11 6,5.9; 12 6,7; 13 -6,7; 14 -6,5.9; 15 -6,4.8; 16 -6,3.7; 17 -6,2.6; 18 -6,-0.4; 19 -6,-1.5; 20 -6,-2.6; 21 -6,-3.7; 22 -6,-4.8; 23 -6,-5.9; 24 -6,-7
MA06-1 = drill 1.016 long: 1 -6.35,0; 2 -3.81,0; 3 -1.27,0; 4 1.27,0; 5 3.81,0; 6 6.35,0
3,3 = hole 3.3: 0,0
QFP50P1600X1600X160-100N = smd 1.475 x 0.3: 1 -7.738,6; 2 -7.738,5.5; 3 -7.738,5; 4 -7.738,4.5; 5 -7.738,4; 6 -7.738,3.5; 7 -7.738,3; 8 -7.738,2.5; 9 -7.738,2; 10 -7.738,1.5; 11 -7.738,1; 12 -7.738,0.5; 13 -7.738,0; 14 -7.738,-0.5; 15 -7.738,-1; 16 -7.738,-1.5; 17 -7.738,-2; 18 -7.738,-2.5; 19 -7.738,-3; 20 -7.738,-3.5; 21 -7.738,-4; 22 -7.738,-4.5; 23 -7.738,-5; 24 -7.738,-5.5; 25 -7.738,-6; 51 7.738,-6; 52 7.738,-5.5; 53 7.738,-5; 54 7.738,-4.5; 55 7.738,-4; 56 7.738,-3.5; 57 7.738,-3; 58 7.738,-2.5; 59 7.738,-2; 60 7.738,-1.5; 61 7.738,-1; 62 7.738,-0.5; 63 7.738,0; 64 7.738,0.5; 65 7.738,1; 66 7.738,1.5; 67 7.738,2; 68 7.738,2.5; 69 7.738,3; 70 7.738,3.5; 71 7.738,4; 72 7.738,4.5; 73 7.738,5; 74 7.738,5.5; 75 7.738,6 | smd 0.3 x 1.475: 26 -6,-7.738; 27 -5.5,-7.738; 28 -5,-7.738; 29 -4.5,-7.738; 30 -4,-7.738; 31 -3.5,-7.738; 32 -3,-7.738; 33 -2.5,-7.738; 34 -2,-7.738; 35 -1.5,-7.738; 36 -1,-7.738; 37 -0.5,-7.738; 38 0,-7.738; 39 0.5,-7.738; 40 1,-7.738; 41 1.5,-7.738; 42 2,-7.738; 43 2.5,-7.738; 44 3,-7.738; 45 3.5,-7.738; 46 4,-7.738; 47 4.5,-7.738; 48 5,-7.738; 49 5.5,-7.738; 50 6,-7.738; 76 6,7.738; 77 5.5,7.738; 78 5,7.738; 79 4.5,7.738; 80 4,7.738; 81 3.5,7.738; 82 3,7.738; 83 2.5,7.738; 84 2,7.738; 85 1.5,7.738; 86 1,7.738; 87 0.5,7.738; 88 0,7.738; 89 -0.5,7.738; 90 -1,7.738; 91 -1.5,7.738; 92 -2,7.738; 93 -2.5,7.738; 94 -3,7.738; 95 -3.5,7.738; 96 -4,7.738; 97 -4.5,7.738; 98 -5,7.738; 99 -5.5,7.738; 100 -6,7.738
SO08 = smd 0.6 x 2.2: 1 -1.905,-2.6; 2 -0.635,-2.6; 3 0.635,-2.6; 4 1.905,-2.6; 5 1.905,2.6; 6 0.635,2.6; 7 -0.635,2.6; 8 -1.905,2.6
MA07-1 = drill 1.016 long: 1 -7.62,0; 2 -5.08,0; 3 -2.54,0; 4 0,0; 5 2.54,0; 6 5.08,0; 7 7.62,0
47346-0001 = smd 0.45 x 1.38: 1 1.3,-4.81; 2 0.65,-4.81; 3 0,-4.81; 4 -0.65,-4.81; 5 -1.3,-4.81 | smd 1.475 x 2.1: 6 -2.453,-4.45; 7 2.453,-4.45 | smd 1.175 x 1.9: 8 0.838,-2.15; 9 -0.838,-2.15 | smd 2.375 x 1.9: 10 2.913,-2.15; 11 -2.913,-2.15
U.FL = smd 2.2 x 0.85: 1 0,1.375; 2 0,-1.375 | smd 1.05 x 1: FEED 1.525,0; NC -1.525,0
ML10 = drill 0.914 octagon: 1 -5.08,-1.27; 2 -5.08,1.27; 3 -2.54,-1.27; 4 -2.54,1.27; 5 0,-1.27; 6 0,1.27; 7 2.54,-1.27; 8 2.54,1.27; 9 5.08,-1.27; 10 5.08,1.27
MA03-1 = drill 1.016 long: 1 -2.54,0; 2 0,0; 3 2.54,0
SHDR2W90P0X350_1X2_750X730X850 = drill 1.45 pad 2.175 square: 1 0,0 | drill 1.45 pad 2.175: 2 3.5,0
R0603 = smd 1 x 1.1: 1 -0.85,0; 2 0.85,0
S64YW = drill 0.813 octagon: A 2.54,1.27; E -2.54,1.27; S 0,-1.27; S@1 0,1.27
PAD-JUMPER-3-NO_YES_SILK = smd 0.635 x 1.27: 1 -0.813,0; 2 0,0; 3 0.813,0
3220-10-0300-00 = smd 0.76 x 2.4: 1 -2.54,-1.95; 2 -2.54,1.95; 3 -1.27,-1.95; 4 -1.27,1.95; 5 0,-1.95; 6 0,1.95; 7 1.27,-1.95; 8 1.27,1.95; 9 2.54,-1.95; 10 2.54,1.95
ESP32SOLO1 = smd 2 x 0.9: 1 -8.5,5.51; 2 -8.5,4.24; 3 -8.5,2.97; 4 -8.5,1.7; 5 -8.5,0.43; 6 -8.5,-0.84; 7 -8.5,-2.11; 8 -8.5,-3.38; 9 -8.5,-4.65; 10 -8.5,-5.92; 11 -8.5,-7.19; 12 -8.5,-8.46; 13 -8.5,-9.73; 14 -8.5,-11; 25 8.5,-11; 26 8.5,-9.73; 27 8.5,-8.46; 28 8.5,-7.19; 29 8.5,-5.92; 30 8.5,-4.65; 31 8.5,-3.38; 32 8.5,-2.11; 33 8.5,-0.84; 34 8.5,0.43; 35 8.5,1.7; 36 8.5,2.97; 37 8.5,4.24; 38 8.5,5.51 | smd 0.9 x 2: 15 -5.715,-12; 16 -4.445,-12; 17 -3.175,-12; 18 -1.905,-12; 19 -0.635,-12; 20 0.635,-12; 21 1.905,-12; 22 3.175,-12; 23 4.445,-12; 24 5.715,-12 | smd 5 x 5: 39 -1,-1.99
CRYSTAL_4.9X1.8 = smd 1.3 x 2.2: 1 -2.1,0; 2 2.1,0

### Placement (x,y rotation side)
C1  56.83,75.88 90 top
C2  52.7,75.88 90 top
C3  65.09,73.66 90 top
C4  67.31,73.66 90 top
C5  50.48,67.63 180 top
C6  50.48,65.41 180 top
C7  70.48,48.26 90 top
C8  72.71,48.26 90 top
C9  74.93,48.26 90 top
C10  77.79,62.87 0 top
C11  75.25,66.67 0 top
C12  77.79,60.64 0 top
C13  67.31,72.07 90 bottom
C14  65.09,72.07 90 bottom
C15  90.81,68.9 180 top
C16  62.55,43.18 90 top
C17  not placed on the board
C18  not placed on the board
C19  not placed on the board
C20  not placed on the board
C21  not placed on the board
C22  not placed on the board
C23  61.59,72.07 90 bottom
C24  58.74,72.07 90 bottom
C25  61.28,64.14 180 bottom
C26  61.28,61.91 180 bottom
C27  64.45,64.14 0 bottom
C28  18.1,97.47 180 top
C29  64.45,61.91 0 bottom
C30  77.79,58.42 0 top
C31  77.79,56.2 0 top
D1  90.81,62.55 0 top
D2  90.81,65.72 270 top
DISPLAY  52.07,31.11 180 top
DISPLAY_TOUCH  33.97,31.11 180 top
FB2  18.1,95.57 0 top
GPS  22.54,85.72 90 top
GPS_DEBUG  25.08,71.75 0 top
H1  5.08,5.08 0 top
H2  5.4,94.93 0 top
H3  94.61,94.93 0 top
H4  94.3,34.29 0 top
H5  42.23,4.76 0 top
IC1  63.18,61.59 270 top
IC4  not placed on the board
IMU-I  78.11,4.76 0 top
IMU-II  58.42,4.76 0 top
J1  99.69,65.41 270 top
J5  13.97,95.57 0 top
MOTOR  92.71,49.21 270 top
MOTOR-L  46.99,93.03 0 top
MOTOR-R  74.61,93.03 0 top
PERIMETER  not placed on the board
POWER(24V)  16.83,4.13 0 top
R1  69.22,29.84 270 top
R2  71.75,29.84 270 top
R3  49.53,35.56 270 top
R4  61.91,47.94 90 top
R5  60.96,9.84 90 top
R6  58.42,9.84 90 top
R7  63.5,9.84 90 top
R8  83.19,9.84 90 top
R9  46.99,35.56 270 top
R10  41.91,35.56 270 top
R11  31.43,35.56 270 top
R12  39.05,35.56 270 top
R13  33.97,35.56 270 top
R14  64.77,43.18 90 top
R15  not placed on the board
R16  not placed on the board
R17  not placed on the board
R18  29.53,95.57 90 top
R19  16.51,75.56 270 top
R20  23.81,95.57 90 top
R21  31.43,68.58 270 bottom
R22  28.89,68.58 270 bottom
R23  21.27,75.56 270 top
R24  23.81,75.56 270 top
R25  21.27,81.28 90 bottom
R26  23.81,81.28 90 bottom
R40  20.64,95.57 270 top
S1_ADR  86.36,9.84 0 top
S2_ADR  66.36,9.84 0 top
SJ1  49.53,86.04 270 top
SJ2  52.07,86.04 270 top
SJ3  77.15,85.72 270 top
SJ4  79.69,85.72 270 top
SJ5  85.41,46.67 180 top
SJ6  85.41,44.13 180 top
SWD  71.12,38.42 90 top
WIFI/BT  14.29,52.07 90 top
Y1  54.93,72.71 180 top

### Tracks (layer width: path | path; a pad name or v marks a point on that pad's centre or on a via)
+3V3  (via drill 0.35)  (4 unrouted)
  Top 0.152: SJ3.1 78.42,86.54 | 78.42,86.54 SJ4.1 | MOTOR-R.8 77.47,94.3 78.42,93.34 78.42,86.54 | SJ1.1 50.8,86.86 | 50.8,86.86 SJ2.1 | MOTOR-L.8 50.8,93.03 50.8,86.86 | 65.18,66.99 IC1.9 65.18,71.34 65.09,71.44 C3.1 | 60.18,66.99 65.18,66.99 | 65.18,66.99 66.99,66.99 67.18,67.18 IC1.5 67.18,71.63 67.31,71.75 C4.1 | DISPLAY.1 62.23,29.53 62.87,28.89 69.11,28.89 | 69.11,28.89 R1.2 69.22,14.29 67.63,12.7 67.63,11.11 | R2.2 71.65,28.89 | 71.65,28.89 69.11,28.89 | 71.65,28.89 72.71,28.89 73.07,29.25 SWD.1 v76.52,35.88 | IMU-II.1 50.8,9.21 52.28,10.69 R6.2 R5.2 R7.2 65.55,10.69 S2_ADR.1 65.55,10.62 66.04,11.11 67.63,11.11 | 67.63,11.11 68.9,11.11 69.32,10.69 70.48,10.69 | 70.48,10.69 IMU-I.1 | 70.48,10.69 R8.2 84.24,10.69 85.09,9.84 S1_ADR.1 | R14.2 64.98,43.81 v68.58,43.81 | v69.22,58.1 v69.22,58.09 IC1.81 76.61,58.09 C30.1 C31.1 | 70.88,64.14 IC1.93 69.22,64.09 v69.22,62.55 70.87,62.55 IC1.90 72.44,62.59 72.71,62.87 C10.1 | IC1.19 60.18,66.99 | 60.18,66.99 59.78,66.59 IC1.28 51.52,66.59 51.44,66.67 | v66.67,58.1 65.68,57.11 IC1.68 65.68,50.2 v68.58,47.31 70.38,47.31 C7.1 C8.1 C9.1 | WIFI/BT.2 10.05,41.7 v12.06,39.69 | R19.2 16.51,72.71 17.46,71.75 GPS_DEBUG.1 | R20.2 R18.2 30.9,96.42 32.38,94.93 v32.38,86.36 | GPS.23 GPS.22 27.3,79.76 v27.3,82.87 | C6.1 51.44,65.51 51.44,66.67 | C5.1 51.44,67.53 51.44,66.67 | SJ5.1 86.22,45.4 | 86.22,45.4 SJ6.1 | MOTOR.8 92.71,45.4 86.22,45.4
  Bottom 0.152: v68.58,43.81 v68.58,47.31 76.52,47.31 | v69.22,62.55 v69.22,58.1 v66.67,58.1 | v12.06,39.69 12.06,69.22 14.61,71.75 GPS_DEBUG.1 18.73,79.59 R25.2 R26.2 27.3,82.13 | v32.38,86.36 28.16,82.13 27.3,82.13 | v27.3,82.87 27.3,82.13 | 76.52,47.31 83.82,47.31 85.72,45.4 92.71,45.4 MOTOR.8 | v76.52,35.88 76.52,47.31
+5V  (4 unrouted)
ANT_VCC1
  Top 0.152: C28.1 18.95,96.2 | 18.95,96.2 FB2.2 | R40.1 20.42,96.2 18.95,96.2
DISP_CS
  Top 0.152: IC1.48 53.42,56.59 52.07,55.24 52.07,50.8 57.78,45.09 57.78,34.29 57.15,33.66 DISPLAY.3
DISP_DC
  Top 0.152: DISPLAY.5 52.07,29.21 52.7,28.57 55.24,28.57 55.88,29.21 55.88,44.13 50.16,49.85 50.16,56.83 51.93,58.59 IC1.44
DISP_MISO  (1 unrouted)
DISP_MOSI  (1 unrouted)
DISP_RS
  Top 0.152: IC1.42 51.66,59.59 48.9,56.83 48.9,49.21 54.61,43.5 DISPLAY.4
DISP_SCK  (1 unrouted)
GND  (via drill 0.35)  (8 unrouted)
  Top 0.152: SJ4.3 SJ3.3 75.11,84.91 74.3,85.72 74.3,87.31 75.88,88.9 75.88,94.93 75.25,95.57 73.34,95.57 MOTOR-R.4 | SJ2.3 SJ1.3 48.44,85.23 47.62,86.04 47.62,87.63 48.26,88.27 48.26,92.39 47.62,93.03 45.72,93.03 MOTOR-L.4 | J1.5 93.69,66.7 93.03,66.04 90.81,66.04 90.37,66.47 D2.1 89.81,68.75 C15.2 | R4.1 v61.91,45.72 62.55,45.09 C16.2 | IMU-II.3 55.88,2.22 56.52,1.59 68.26,1.59 | 68.26,1.59 74.93,1.59 75.56,2.22 | S2_ADR.3 67.17,8.08 68.26,6.99 68.26,1.59 | IMU-I.3 75.56,2.22 | 75.56,2.22 76.2,1.59 87,1.59 87.95,2.54 87.95,6.99 87.17,7.76 S1_ADR.3 | IC1.29 57.09,66.09 v57.78,65.41 v61.91,65.41 | WIFI/BT.38 8.78,76.09 12.41,79.72 GPS.13 | GPS.12 15.51,91.76 14.29,91.76 13.97,92.08 J5.2 J5.1 14.5,97.47 C28.2 | C10.2 C12.2 C30.2 C31.2 | 49.53,65.3 C6.2 C5.2 | C3.2 C4.2 | SJ6.3 SJ5.3
  Bottom 0.152: v61.91,65.41 62.13,65.19 C25.2 63.5,64.14 | 63.5,64.14 C27.2 | C29.2 63.5,62.02 | 63.5,62.02 63.5,64.14 | C26.2 62.23,62.02 63.5,62.02
  pour Top: -0.32,100.33 100.97,100.33 100.97,-0.64 101.28,-0.95 -0.64,-0.95 -0.95,-1.27 -0.95,100.33
  pour Bottom: -0.95,100.33 100.65,100.33 100.97,100.01 100.97,-0.64 101.28,-0.95 -0.95,-0.95
GPS_ANT2
  Top 0.152: J5.FEED 16.83,95.57 | 16.83,95.57 FB2.1 | GPS.11 16.64,95.38 16.83,95.57
GPS_PPS
  Top 0.152: WIFI/BT.31 17.67,62.44 21.59,66.36 33.66,66.36 | 33.66,66.36 33.66,81.92 27.3,88.27 27.3,91.69 GPS.3 | IC1.34 42.45,63.59 39.69,66.36 33.66,66.36
GPS_RXD
  Top 0.152: GPS.21 26.24,78.53 31.43,73.34 GPS_DEBUG.6
  Bottom 0.152: R21.1 GPS_DEBUG.6
GPS_SCL  (via drill 0.35)
  Top 0.152: WIFI/BT.36 11.32,67.83 13.02,69.53 v16.19,69.53 | GPS.19 24.04,77.7 v23.81,77.47 R24.1
  Bottom 0.152: R26.1 v23.81,77.47 23.18,77.47 22.54,76.83 22.54,70.17 21.91,69.53 v16.19,69.53
GPS_SDA  (via drill 0.35)
  Top 0.152: WIFI/BT.33 15.13,62.44 20,67.31 20,75.88 20.54,76.42 R23.1 v21.27,78.11 22.54,78.11 22.94,78.5 GPS.18
  Bottom 0.152: R25.1 v21.27,78.11
GPS_TXD
  Top 0.152: GPS.20 25.14,78.68 28.89,74.93 GPS_DEBUG.5
  Bottom 0.152: R22.1 GPS_DEBUG.5
ML_MODE1
  Top 0.152: SJ1.2 48.58,86.04 48.26,86.36 48.26,87.31 49.53,88.58 MOTOR-L.7
ML_MODE2
  Top 0.152: SJ2.2 53.02,86.04 53.34,86.36 53.34,87.31 52.07,88.58 MOTOR-L.9
ML_MON_CUR  (via drill 0.35)
  Top 0.152: MOTOR-L.6 46.99,95.89 47.94,96.84 58.42,96.84 63.5,91.76 63.5,85.09 v63.5,83.19 | IC1.14 62.68,76.97 v63.5,77.79
  Bottom 0.152: v63.5,77.79 v63.5,83.19
ML_NFAULT
  Top 0.152: MOTOR-L.10 55.56,94.3 59.68,90.18 IC1.20
ML_PHASE
  Top 0.152: IC1.21 59.18,78.3 54.61,82.87 48.9,82.87 46.99,84.77 MOTOR-L.5
MOT_EN
  Top 0.152: IC1.80 72.58,57.59 75.88,54.29 MOTOR.1
MOT_MODE1
  Top 0.152: SJ5.2 85.41,47.62 85.72,47.94 86.68,47.94 87.95,46.67 MOTOR.7
MOT_MODE2
  Top 0.152: SJ6.2 85.41,43.18 85.72,42.86 86.68,42.86 87.95,44.13 MOTOR.9
MOT_MON_CUR  (via drill 0.35)
  Top 0.152: IC1.16 61.68,74.53 v61.28,74.93
  Bottom 0.152: MOTOR.6 92.71,50.48 76.83,50.48 72.07,55.24 61.91,55.24 56.2,60.96 56.2,66.99 56.2,67.31 56.2,73.66 57.47,74.93 v61.28,74.93
MOT_NFAULT
  Top 0.152: IC1.77 72.17,56.09 80.01,48.26 89.85,48.26 90.17,47.94 95.25,47.94 95.89,47.31 95.89,44.45 95.57,44.13 MOTOR.10
MOT_NSLEEP
  Top 0.152: IC1.79 72.44,57.09 77.79,51.75 MOTOR.3
MOT_PHASE
  Top 0.152: IC1.78 72.31,56.59 79.69,49.21 MOTOR.5
MOTOR_EN
  Bottom 0.152: MOTOR-L.1 41.91,88.9 42.55,88.27 68.9,88.27 69.53,88.9 MOTOR-R.1
MOTOR_NSLEEP
  Bottom 0.152: MOTOR-L.3 44.45,89.85 45.09,89.22 67.94,89.22 67.94,92.39 68.58,93.03 70.8,93.03 MOTOR-R.3
MR_MODE1
  Top 0.152: SJ3.2 76.2,85.72 75.88,86.04 75.88,87 77.15,88.27 MOTOR-R.7
MR_MODE2
  Top 0.152: SJ4.2 80.64,85.72 80.96,86.04 80.96,87 79.69,88.27 MOTOR-R.9
MR_MON_CUR
  Top 0.152: IC1.15 62.18,78.06 73.34,89.22 73.34,93.03 MOTOR-R.6
MR_NFAULT
  Top 0.152: MOTOR-R.10 81.6,94.3 83.5,92.39 83.5,84.14 82.87,83.5 79.69,83.5 69.18,72.99 IC1.1
MR_PHASE
  Top 0.152: MOTOR-R.5 74.61,89.22 68.68,83.29 IC1.2
N$1
  Top 0.152: IC1.60 61.68,50.08 61.91,49.85 R4.2
N$2  (via drill 0.35)
  Top 0.152: D1.2 93.34,62.55 93.66,62.87 v93.66,63.5 93.66,63.82 93.95,64.11 J1.1 | v93.03,67.31 91.81,67.31 D2.4 91.81,68.75 C15.1
  Bottom 0.152: v93.03,67.31 95.57,67.31 95.89,66.99 95.89,63.82 95.57,63.5 v93.66,63.5
N$3  (1 unrouted)
N$4  (1 unrouted)
N$5
  Top 0.152: R23.2 GPS_DEBUG.2
N$6  (1 unrouted)
N$7  (1 unrouted)
N$8  (1 unrouted)
N$9  (1 unrouted)
N$10  (1 unrouted)
N$11  (1 unrouted)
N$12
  Top 0.152: R24.2 GPS_DEBUG.3
N$13
  Top 0.152: GPS.1 29.54,94.7 R18.1
N$14
  Top 0.152: GPS.8 19.98,91.76 20.64,91.76 21.91,93.03 21.91,93.66 22.96,94.72 R20.1
N$15
  Top 0.152: GPS.14 16.64,76.55 R19.1
N$29
  Top 0.152: GPS.9 18.84,93.45 20.11,94.72 R40.2
PA7_XIN32
  Top 0.152: IC1.24 57.68,70.91 57.03,71.56 Y1.1 56.83,72.9 C1.1
PA8_XOUT32
  Top 0.152: IC1.25 57.18,70.45 56.83,70.8 53.34,70.8 52.83,71.31 Y1.2 52.7,72.83 C2.1
PA09_UART_RXD_0  (via drill 0.35)
  Top 0.152: v56.52,50.16 58.1,50.16 58.68,50.74 IC1.54
  Bottom 0.152: v56.52,50.16 40.01,50.16 28.89,61.28 R22.2
PA10_UART_TXD_0  (via drill 0.35)
  Top 0.152: IC1.46 52.52,57.59 v52.07,57.15
  Bottom 0.152: R21.2 31.43,63.82 38.1,57.15 v52.07,57.15
PA20_PERIMETER_SENDER  (2 unrouted)
PA21_USB_N
  Top 0.152: IC1.94 88.76,64.59 89.22,64.14 90.49,64.14 91.12,64.77 D2.3 91.82,64.75 J1.2
PA22_USB_P
  Top 0.152: IC1.95 88.89,65.09 89.22,64.77 D2.2 90.49,64.77 91.12,65.41 J1.3
PB01_SPI_4_SCK  (via drill 0.35)
  Top 0.152: R9.1 v46.99,37.78 | IC1.47 53.28,57.09 51.44,55.24 51.44,50.48 57.15,44.77 v57.15,37.78 | v39.05,37.78 R12.1
  Bottom 0.152: v57.15,37.78 v46.99,37.78 v39.05,37.78
PB6_SWDIO_TMS
  Top 0.152: IC1.57 60.18,38.56 62.87,35.88 SWD.2 69.17,30.74 R1.1
PB7_SWCLK_TCK
  Top 0.152: 71.12,37.15 71.12,33.66 71.75,33.02 R2.1 | 71.12,37.15 71.12,44.13 70.17,45.09 65.72,45.09 63.18,47.62 IC1.63 | SWD.4 71.12,37.15
PB10_SPI_4_MOSI  (via drill 0.35)
  Top 0.152: IC1.43 51.79,59.09 49.53,56.83 49.53,49.53 55.24,43.81 v55.24,38.73 | R3.1 v49.53,38.73 | v33.97,38.73 R13.1
  Bottom 0.152: v55.24,38.73 v49.53,38.73 v33.97,38.73
PB11_SPI_4_MISO  (via drill 0.35)
  Top 0.152: IC1.45 52.06,58.09 50.8,56.83 50.8,50.16 56.52,44.45 v56.52,39.69 | R11.1 31.43,38.73 32.38,39.69 41.91,39.69 | v51.75,39.69 41.91,39.69 | R10.1 41.91,39.69
  Bottom 0.152: v56.52,39.69 v51.75,39.69
PD25_UART_RXD_2
  Top 0.152: WIFI/BT.28 21.48,62.44 22.14,63.09 IC1.35
PD26_UART_TXD_2
  Top 0.152: WIFI/BT.27 22.75,62.16 23.18,62.59 IC1.36
SENSOR_1_CS
  Top 0.152: R8.1 IMU-I.6
SENSOR_1_SA_0
  Top 0.152: S1_ADR.2 86.36,8.26 85.72,7.62 IMU-I.7
SENSOR_2_CS
  Top 0.152: R7.1 IMU-II.6
SENSOR_2_SA_0
  Top 0.152: S2_ADR.2 66.36,8.26 66.04,7.94 IMU-II.7
SENSOR_3V3  (1 unrouted)
SENSOR_SCL  (via drill 0.35)  (1 unrouted)
  Top 0.152: IC1.55 59.18,47.18 59.69,46.67 59.69,37.78 63.18,34.29 v65.72,34.29
  Bottom 0.152: v65.72,34.29 65.72,23.18 58.42,15.88 IMU-II.4 58.42,2.54 59.87,1.09 76.97,1.09 78.11,2.22 IMU-I.4
SENSOR_SDA  (via drill 0.35)  (1 unrouted)
  Top 0.152: IC1.64 63.68,47.76 65.41,46.04 v66.67,46.04
  Bottom 0.152: v66.67,46.04 66.67,22.86 60.96,17.14 IMU-II.5 60.96,2.54 61.59,1.91 76.2,1.91 76.83,2.54 76.83,6.67 77.47,7.3 80.01,7.3 80.64,6.67 IMU-I.5
TARGET_RESET
  Top 0.152: IC1.58 60.68,42.19 61.91,40.96 65.09,40.96 | 65.09,40.96 SWD.10 | C16.1 R14.1 65.09,42.01 65.09,40.96
TOUCH_CLK
  Top 0.152: DISPLAY_TOUCH.1 R12.2
TOUCH_CS  (via drill 0.35)
  Top 0.152: IC1.50 53.86,55.59 53.22,54.96 53.22,51.55 59.05,45.72 v59.05,36.51
  Bottom 0.152: DISPLAY_TOUCH.2 36.51,35.56 37.47,36.51 v59.05,36.51
TOUCH_IRQ  (via drill 0.35)
  Top 0.152: IC1.49 53.55,56.09 52.7,55.24 52.7,51.12 58.42,45.4 v58.42,40.64 | DISPLAY_TOUCH.5 v28.89,38.73
  Bottom 0.152: v58.42,40.64 30.8,40.64 v28.89,38.73
TOUCH_MISO
  Top 0.152: DISPLAY_TOUCH.4 R11.2
TOUCH_MOSI
  Top 0.152: DISPLAY_TOUCH.3 R13.2
VCCINT  (via drill 0.35)  (1 unrouted)
  Top 0.152: IC1.22 58.68,67.68 58.74,67.63 v59.05,67.63 | v61.59,67.63 60.96,67.63 60.68,67.91 IC1.18 | IC1.4 67.68,67.89 v67.94,67.63 67.94,65.41 | 67.94,60.64 67.94,65.59 IC1.96 72.58,65.59 73.66,66.67 C11.1 | 67.94,60.64 67.99,60.59 IC1.86 76.89,60.59 C12.1 | IC1.39 58.55,61.09 v59.05,61.59 | IC1.76 68.55,55.59 67.94,56.2 67.94,60.64
  Bottom 0.152: v61.59,67.63 v59.05,67.63 59.05,64.14 | v61.59,67.63 65.09,67.63 | 65.09,67.63 67.31,67.63 | 67.31,67.63 v67.94,67.63 | 59.05,64.14 v59.05,61.59 59.37,61.91 C26.1 | C24.1 C23.1 v61.59,67.63 | C14.1 65.09,67.63 | C13.1 67.31,67.63 | C25.1 59.05,64.14 | 65.09,67.63 65.3,67.41 C27.1 C29.1

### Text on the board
Measures: Measurements in inches

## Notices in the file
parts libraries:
SparkFun-Connectors: Licensing: Creative Commons ShareAlike 4.0 International - https://creativecommons.org/licenses/by-sa/4.0
microbuilder: This work is placed in the public domain, and may be freely used for commercial and non-commercial work with the following conditions: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
